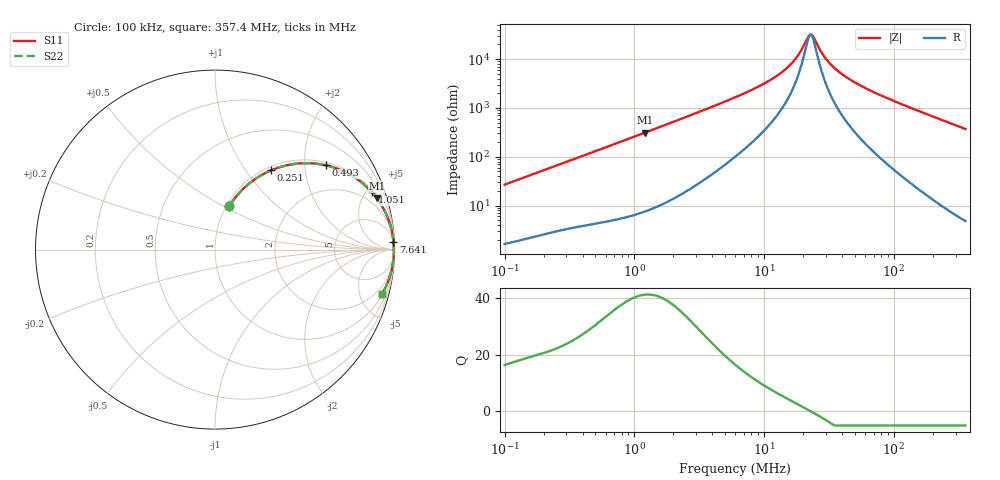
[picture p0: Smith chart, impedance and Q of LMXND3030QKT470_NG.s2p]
! LMXND3030QKT470_NG  S-PARAMETER MODEL  ( Standard Model )
! Model Generated by TAIYO YUDEN Corporation (https://www.yuden.co.jp/en/)
! Version 1.0
! TAIYO YUDEN Control No. 20250523
! Copyright(c) 2025 TAIYO YUDEN CO.,LTD. All Rights Reserved.
! Product Description (link to TY-COMPAS)
! https://ds.yuden.co.jp/TYCOMPAS/or/detail?pn=LMXND3030QKT470MNG&u=M
! Products Name : Inductors
! Characteristics :
!  Inductance : 47 [uH] , SRF(min) : 17 [MHz] , DC Resistance(max) : 1.32 [Ohm]
!  Rated Current : Saturation  325 [mA] , Temp Rise  350 [mA] (40 [degC])
!  Case Size : 3.0 x 3.0 / 0.118 x 0.118 [mm/inch] , Thickness : 1.5 / 0.059 [mm/inch]
!  (Conditions: Temperature = 25 [degC] , DC Bias Current = 0 [A])
! External Node Assignments :
!  1  o---GGG---o  2
! GND o---------o GND
! Frequency Range : 0.1MHz  -  357.398349MHz  [ 402 STEP ]
# MHz S RI R 50
! Freq[MHz].  S11 Real  S11 Imag  S21 Real  S21 Imag  S12 Real  S12 Imag  S22 Real  S22 Imag
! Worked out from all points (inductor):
!   401 points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, 100 kHz to 357.4 MHz, reference 50 ohm
!   read as one part in series: L = 42.6 uH near 104.2 kHz
!   highest Q = 41.2 at 1.213 MHz (marker M1), where L = 41.1 uH
!   self-resonance near 22.59 MHz
!   S11 on the Smith chart (normalised r, x): 100 kHz: 1.03, +0.54; 251 kHz: 1.06, +1.32; 493 kHz: 1.08, +2.56; 1.051 MHz: 1.13, +5.43; 7.641 MHz: 4, +44; 357.4 MHz: 1.10, -7.41
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0.1  0.0804 0.243  0.9196 -0.243  0.9196 -0.243  0.0804 0.243
0.160069  0.1665 0.3474  0.8335 -0.3474  0.8335 -0.3474  0.1665 0.3474
0.251032  0.312 0.4413  0.688 -0.4413  0.688 -0.4413  0.312 0.4413
0.393689  0.5124 0.4817  0.4876 -0.4817  0.4876 -0.4817  0.5124 0.4817
0.49302  0.6173 0.4698  0.3827 -0.4698  0.3827 -0.4698  0.6173 0.4698
0.727176  0.7733 0.4052  0.2267 -0.4052  0.2267 -0.4052  0.7733 0.4052
1.050827  0.8744 0.3193  0.1256 -0.3193  0.1256 -0.3193  0.8744 0.3193
1.212583  0.9018 0.2857  0.0982 -0.2857  0.0982 -0.2857  0.9018 0.2857
1.549909  0.9363 0.2322  0.0637 -0.2322  0.0637 -0.2322  0.9363 0.2322
2.921968  0.9791 0.1277  0.0209 -0.1277  0.0209 -0.1277  0.9791 0.1277
6.101817  0.9929 0.0587  0.00713 -0.0587  0.00713 -0.0587  0.9929 0.0587
7.641363  0.9944 0.045  0.00559 -0.045  0.00559 -0.045  0.9944 0.045
11.27056  0.9959 0.0261  0.00409 -0.0261  0.00409 -0.0261  0.9959 0.0261
14.70358  0.9965 0.0156  0.00354 -0.0156  0.00354 -0.0156  0.9965 0.0156
18.04064  0.9967 0.00823  0.00329 -0.00823  0.00329 -0.00823  0.9967 0.00823
22.13506  0.9969 0.0012  0.00314 -0.0012  0.00314 -0.0012  0.9969 0.0012
23.53582  0.9969 -0.0009  0.00311 0.0009  0.00311 0.0009  0.9969 -0.0009
29.47413  0.9969 -0.00869  0.0031 0.00869  0.0031 0.00869  0.9969 -0.00869
36.91074  0.9968 -0.017  0.00324 0.017  0.00324 0.017  0.9968 -0.017
53.33896  0.9961 -0.0326  0.00392 0.0326  0.00392 0.0326  0.9961 -0.0326
92.65788  0.9929 -0.0652  0.00708 0.0652  0.00708 0.0652  0.9929 -0.0652
357.3983  0.9294 -0.2498  0.0706 0.2498  0.0706 0.2498  0.9294 -0.2498
